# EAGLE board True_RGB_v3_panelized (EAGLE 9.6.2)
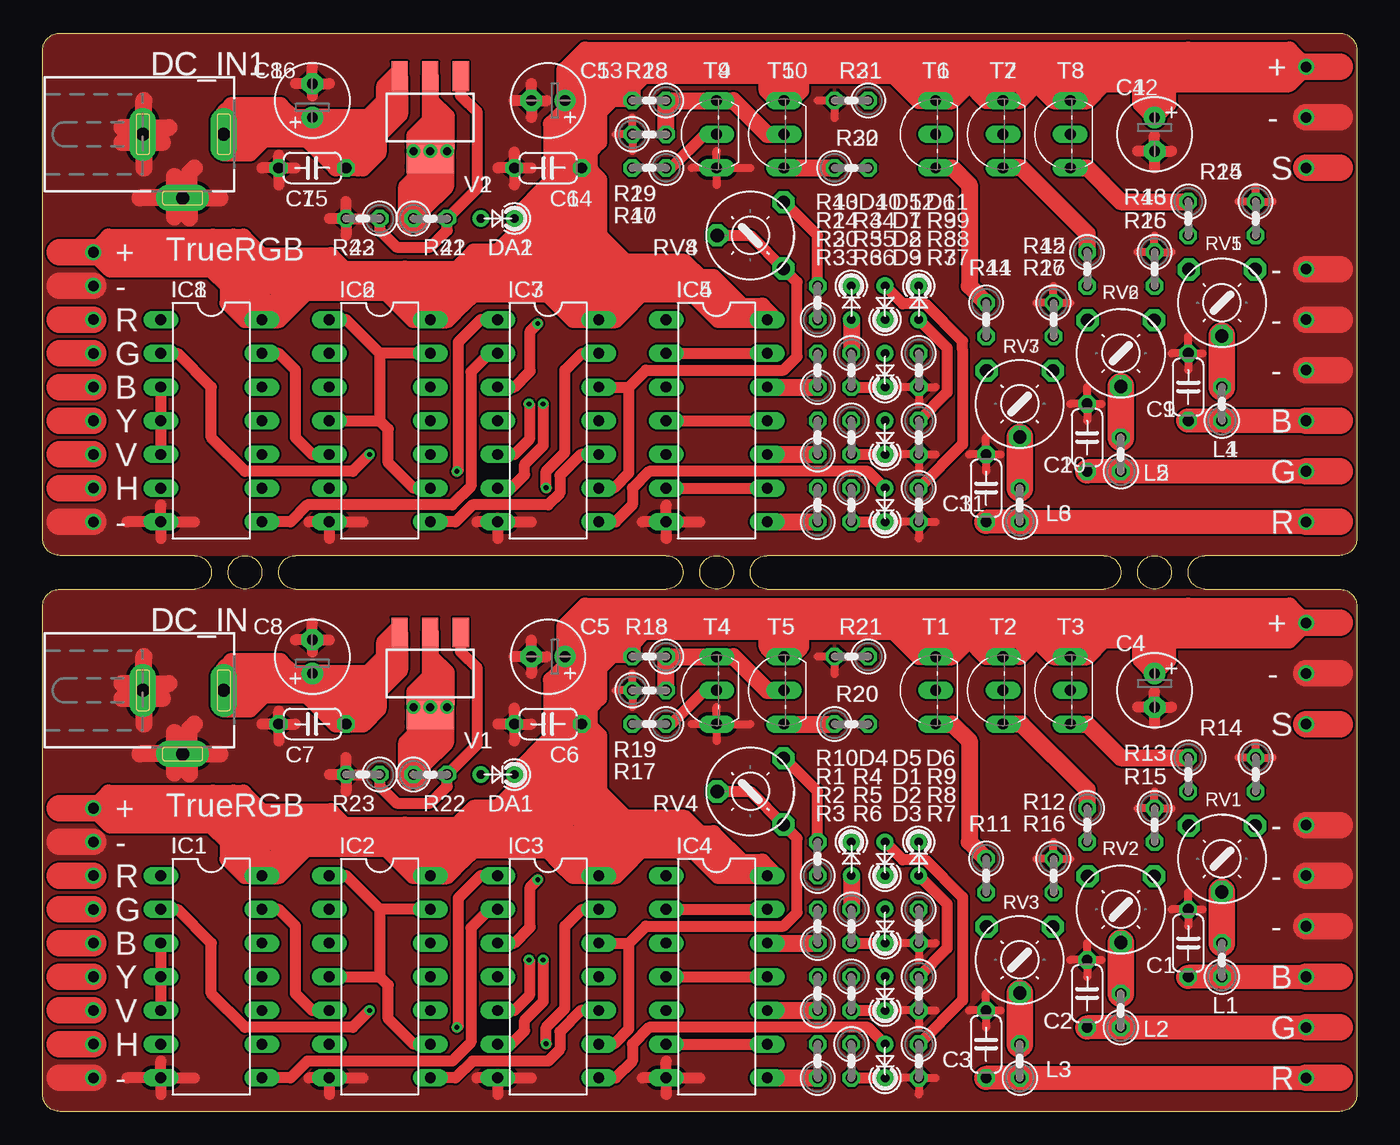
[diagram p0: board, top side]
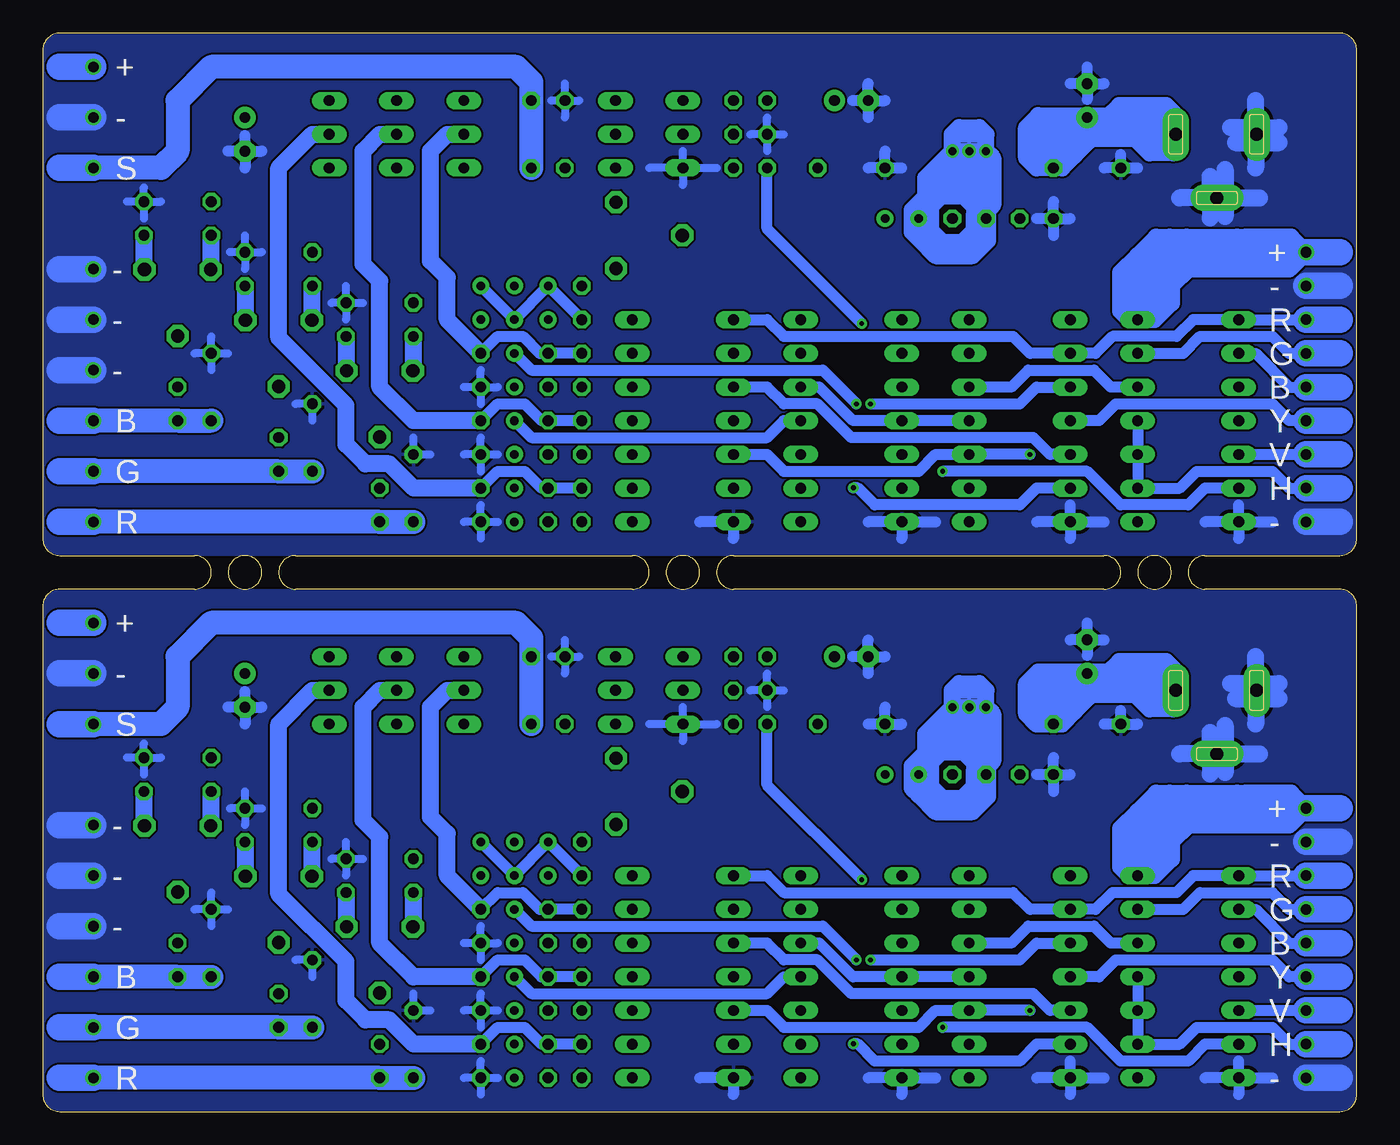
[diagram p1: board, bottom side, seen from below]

Size 99.06 x 81.28 mm. Coordinates in mm from the lower left corner, seen from the top.
Outline: 97.79,0 1.27,0 arc-90 0,1.27 0,38.1 arc-90 1.27,39.37 11.43,39.37 arc180 11.43,41.91 1.27,41.91 arc-90 0,43.18 0,80.01 arc-90 1.27,81.28 97.79,81.28 arc-90 99.06,80.01 99.06,43.18 arc-90 97.79,41.91 87.63,41.91 arc180 87.63,39.37 97.79,39.37 arc-90 99.06,38.1 99.06,1.27 arc-90 97.79,0
Outline: 19.05,39.37 46.99,39.37 arc180 46.99,41.91 19.05,41.91 arc180 19.05,39.37
Outline: 54.61,39.37 80.01,39.37 arc180 80.01,41.91 54.61,41.91 arc180 54.61,39.37
Outline: 15.24,39.37 arc-180 15.24,41.91 arc-180 15.24,39.37
Outline: 83.82,41.91 arc-180 83.82,39.37 arc-180 83.82,41.91
Outline: 50.8,41.91 arc-180 50.8,39.37 arc-180 50.8,41.91
Copper layers (1*16): Top 0.035mm / dielectric 1.5mm / Bottom 0.035mm
Design rules "default *": minimum track width 6mil, minimum drill 0.35mm, track to track 6mil, track to pad 6mil, pad to pad 6mil, via to via 6mil, smd to smd 6mil, copper to edge 2mil, drill to drill 6mil, minimum pad ring 10mil, minimum via ring 8mil, stop-mask expansion 4mil, vias tented up to drill 20mil, thermal gap 10mil
Net classes: 1 power: width 0.66 mm, clearance 0.254 mm

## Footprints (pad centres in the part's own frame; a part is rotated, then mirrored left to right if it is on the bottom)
C050-024X044 = drill 0.813 octagon: 1 -2.54,0; 2 2.54,0
E2,5-6 = drill 0.813 pad 1.6: + -1.27,0 | drill 0.813 pad 1.6 octagon: - 1.27,0
D4148-2 = drill 0.65 pad 1.27: A 1.27,0; C -1.27,0
DCJ0202 = drill 1 pad 2 long: 1 0,3.1; 2 4.8,0; 3 0,-3
DIL14 = drill 0.813 long: 1 -7.62,-3.81; 2 -5.08,-3.81; 3 -2.54,-3.81; 4 0,-3.81; 5 2.54,-3.81; 6 5.08,-3.81; 7 7.62,-3.81; 8 7.62,3.81; 9 5.08,3.81; 10 2.54,3.81; 11 0,3.81; 12 -2.54,3.81; 13 -5.08,3.81; 14 -7.62,3.81
0207/2V = drill 0.813 octagon: 1 -1.27,0; 2 1.27,0
6MM = drill 1 pad 1.676 octagon: A -2.5,-2.5; E 2.5,-2.5; S 0,2.5
TO92-EBC = drill 0.813 long: B 0,-1.27; C 2.54,-1.27; E -2.54,-1.27
SOT223 = smd 1.219 x 2.235: 1 -2.311,-3.099; 2 0,-3.099; 3 2.311,-3.099 | smd 3.6 x 2.2: TAB 0,3.099

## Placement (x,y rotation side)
C1  47  [C050-024X044]  86.36,12.7 90 top
C2  47  [C050-024X044]  78.74,8.89 90 top
C3  47  [C050-024X044]  71.12,5.08 90 top
C4  10uF  [E2,5-6]  83.82,31.75 270 top
C5  100uF  [E2,5-6]  38.1,34.29 180 top
C6  0.1uF  [C050-024X044]  38.1,29.21 180 top
C7  0.1uF  [C050-024X044]  20.32,29.21 180 top
C8  100uF  [E2,5-6]  20.32,34.29 90 top
C9  47  [C050-024X044]  86.36,54.61 90 top
C10  47  [C050-024X044]  78.74,50.8 90 top
C11  47  [C050-024X044]  71.12,46.99 90 top
C12  10uF  [E2,5-6]  83.82,73.66 270 top
C13  100uF  [E2,5-6]  38.1,76.2 180 top
C14  0.1uF  [C050-024X044]  38.1,71.12 180 top
C15  0.1uF  [C050-024X044]  20.32,71.12 180 top
C16  100uF  [E2,5-6]  20.32,76.2 90 top
D1  1N4148AS  [D4148-2]  63.5,13.97 90 top
D2  1N4148AS  [D4148-2]  63.5,8.89 90 top
D3  1N4148AS  [D4148-2]  63.5,3.81 90 top
D4  1N4148AS  [D4148-2]  60.96,19.05 270 top
D5  1N4148AS  [D4148-2]  63.5,19.05 90 top
D6  1N4148AS  [D4148-2]  66.04,19.05 270 top
D7  1N4148AS  [D4148-2]  63.5,55.88 90 top
D8  1N4148AS  [D4148-2]  63.5,50.8 90 top
D9  1N4148AS  [D4148-2]  63.5,45.72 90 top
D10  1N4148AS  [D4148-2]  60.96,60.96 270 top
D11  1N4148AS  [D4148-2]  66.04,60.96 270 top
D12  1N4148AS  [D4148-2]  63.5,60.96 90 top
DA1  BAT42  [D4148-2]  34.29,25.4 180 top
DA2  BAT42  [D4148-2]  34.29,67.31 180 top
DC_IN  DCJ0202  [DCJ0202]  10.54,31.75 270 top
DC_IN1  DCJ0202  [DCJ0202]  10.54,73.66 270 top
IC1  7427 ЛЕ4  [DIL14]  12.7,10.16 270 top
IC2  7400 ЛА3  [DIL14]  25.4,10.16 270 top
IC3  7400 ЛА3  [DIL14]  38.1,10.16 270 top
IC4  7404 ЛН1  [DIL14]  50.8,10.16 270 top
IC5  7404 ЛН1  [DIL14]  50.8,52.07 270 top
IC6  7400 ЛА3  [DIL14]  25.4,52.07 270 top
IC7  7400 ЛА3  [DIL14]  38.1,52.07 270 top
IC8  7427 ЛЕ4  [DIL14]  12.7,52.07 270 top
L1  0.56uH  [0207/2V]  88.9,11.43 90 top
L2  0.56uH  [0207/2V]  81.28,7.62 90 top
L3  0.56uH  [0207/2V]  73.66,3.81 90 top
L4  0.56uH  [0207/2V]  88.9,53.34 90 top
L5  0.56uH  [0207/2V]  81.28,49.53 90 top
L6  0.56uH  [0207/2V]  73.66,45.72 90 top
R1  2.1k  [0207/2V]  58.42,13.97 90 top
R2  2.1k  [0207/2V]  58.42,8.89 90 top
R3  2.1k  [0207/2V]  58.42,3.81 90 top
R4  330  [0207/2V]  60.96,13.97 270 top
R5  330  [0207/2V]  60.96,8.89 270 top
R6  330  [0207/2V]  60.96,3.81 270 top
R7  5.1K  [0207/2V]  66.04,3.81 270 top
R8  5.1K  [0207/2V]  66.04,8.89 270 top
R9  5.1K  [0207/2V]  66.04,13.97 270 top
R10  130  [0207/2V]  58.42,19.05 90 top
R11  100  [0207/2V]  71.12,17.78 270 top
R12  100  [0207/2V]  78.74,21.59 270 top
R13  100  [0207/2V]  86.36,25.4 270 top
R14  75  [0207/2V]  91.44,25.4 270 top
R15  75  [0207/2V]  83.82,21.59 270 top
R16  75  [0207/2V]  76.2,17.78 270 top
R17  1K  [0207/2V]  45.72,29.21 180 top
R18  1K  [0207/2V]  45.72,34.29 180 top
R19  1K  [0207/2V]  45.72,31.75 0 top
R20  47  [0207/2V]  60.96,29.21 0 top
R21  560  [0207/2V]  60.96,34.29 180 top
R22  220  [0207/2V]  29.21,25.4 0 top
R23  680  [0207/2V]  24.13,25.4 180 top
R24  2.1k  [0207/2V]  58.42,55.88 90 top
R25  75  [0207/2V]  91.44,67.31 270 top
R26  75  [0207/2V]  83.82,63.5 270 top
R27  75  [0207/2V]  76.2,59.69 270 top
R28  1K  [0207/2V]  45.72,76.2 180 top
R29  1K  [0207/2V]  45.72,73.66 0 top
R30  2.1k  [0207/2V]  58.42,50.8 90 top
R31  560  [0207/2V]  60.96,76.2 180 top
R32  47  [0207/2V]  60.96,71.12 0 top
R33  2.1k  [0207/2V]  58.42,45.72 90 top
R34  330  [0207/2V]  60.96,55.88 270 top
R35  330  [0207/2V]  60.96,50.8 270 top
R36  330  [0207/2V]  60.96,45.72 270 top
R37  5.1K  [0207/2V]  66.04,45.72 270 top
R38  5.1K  [0207/2V]  66.04,50.8 270 top
R39  5.1K  [0207/2V]  66.04,55.88 270 top
R40  1K  [0207/2V]  45.72,71.12 180 top
R41  220  [0207/2V]  29.21,67.31 0 top
R42  680  [0207/2V]  24.13,67.31 180 top
R43  130  [0207/2V]  58.42,60.96 90 top
R44  100  [0207/2V]  71.12,59.69 270 top
R45  100  [0207/2V]  78.74,63.5 270 top
R46  100  [0207/2V]  86.36,67.31 270 top
RV1  200  [6MM]  88.9,19.05 180 top
RV2  200  [6MM]  81.28,15.24 180 top
RV3  200  [6MM]  73.66,11.43 180 top
RV4  200  [6MM]  53.34,24.13 90 top
RV5  200  [6MM]  88.9,60.96 180 top
RV6  200  [6MM]  81.28,57.15 180 top
RV7  200  [6MM]  73.66,53.34 180 top
RV8  200  [6MM]  53.34,66.04 90 top
T1  4401  [TO92-EBC]  66.04,31.75 90 top
T2  4401  [TO92-EBC]  71.12,31.75 90 top
T3  4401  [TO92-EBC]  76.2,31.75 90 top
T4  4401  [TO92-EBC]  49.53,31.75 90 top
T5  4401  [TO92-EBC]  54.61,31.75 90 top
T6  4401  [TO92-EBC]  66.04,73.66 90 top
T7  4401  [TO92-EBC]  71.12,73.66 90 top
T8  4401  [TO92-EBC]  76.2,73.66 90 top
T9  4401  [TO92-EBC]  49.53,73.66 90 top
T10  4401  [TO92-EBC]  54.61,73.66 90 top
V1  LM1117IMPX-ADJ  [SOT223]  29.21,33.02 180 top
V2  LM1117IMPX-ADJ  [SOT223]  29.21,74.93 180 top

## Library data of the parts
C1-C16 = rcl; SPICEPREFIX: C
D1-D12 DA1 DA2 RV1-RV8 = 27C322
DC_IN DC_IN1 = power_jack; OC_FARNELL: unknown; OC_NEWARK: unknown
IC1-IC8 = 74xx-eu
L1-L6 = rcl; SPICEPREFIX: L
R1-R46 = rcl; SPICEPREFIX: R
T1-T10 = transistor-neu-to92
V1 V2 = lm1117

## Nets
B: IC1.2 IC2.10 IC4.5
B1: IC5.5 IC6.10 IC8.2
BLUE: C1.1 L1.1
BLUE1: C9.1 L4.1
G: IC1.13 IC2.5 IC4.3
G1: IC5.3 IC6.5 IC8.13
GND: C1.2 C2.2 C3.2 C4.- C5.- C6.2 C7.2 C8.- DC_IN.2 DC_IN.3 IC1.7 IC2.7 IC3.7 IC4.7 R7.2 R8.2 R9.2 R14.1 R15.1 R16.1 R19.1 R21.2 R23.2 T4.E
GND1: C9.2 C10.2 C11.2 C12.- C13.- C14.2 C15.2 C16.- DC_IN1.2 DC_IN1.3 IC5.7 IC6.7 IC7.7 IC8.7 R25.1 R26.1 R27.1 R29.1 R31.2 R37.2 R38.2 R39.2 R42.2 T9.E
GREEN: C2.1 L2.1
GREEN1: C10.1 L5.1
H: IC1.9 IC1.10 IC1.11
H1: IC8.9 IC8.10 IC8.11
N$1: D3.C R6.2
N$2: D2.C R5.2
N$3: D1.C R4.2
N$4: L1.2 RV1.S
N$5: IC1.12 IC2.12
N$6: IC1.8 IC3.2
N$7: L2.2 RV2.S
N$8: D5.A R3.2 R6.1 R7.1 T3.B
N$9: D6.A R2.2 R5.1 R8.1 T2.B
N$10: D4.A R1.2 R4.1 R9.1 T1.B
N$11: L3.2 RV3.S
N$12: R14.2 RV1.A
N$13: R15.2 RV2.A
N$14: R16.2 RV3.A
N$15: R11.1 T1.E
N$16: R12.2 RV2.E
N$17: R11.2 RV3.E
N$18: R12.1 T2.E
N$19: IC2.3 IC3.5
N$20: IC2.6 IC3.13
N$21: IC2.8 IC3.10
N$22: D1.A IC3.6
N$23: D2.A IC3.11
N$24: D3.A IC3.8
N$25: IC4.2 IC4.13
N$26: IC4.4 IC4.11
N$27: IC4.6 IC4.9
N$28: IC4.12 R1.1
N$29: IC4.10 R2.1
N$30: IC4.8 R3.1
N$31: IC3.3 R17.2
N$32: R22.2 R23.1 V1.1
N$33: IC1.6 IC3.1
N$34: R17.1 T4.B
N$35: DA1.A R22.1 V1.2 V1.TAB
N$36: D4.C D5.C D6.C R10.1
N$37: R10.2 RV4.E
N$38: IC2.11 IC3.4 IC3.9 IC3.12 RV4.A RV4.S
N$39: R13.1 T3.E
N$40: R13.2 RV1.E
N$41: D12.A R33.2 R36.1 R37.1 T8.B
N$42: D11.A R30.2 R35.1 R38.1 T7.B
N$43: D10.A R24.2 R34.1 R39.1 T6.B
N$44: R28.1 R29.2 T9.C T10.B
N$45: R32.1 T10.E
N$46: L4.2 RV5.S
N$47: L5.2 RV6.S
N$48: L6.2 RV7.S
N$49: R25.2 RV5.A
N$50: R26.2 RV6.A
N$51: R27.2 RV7.A
N$52: R45.2 RV6.E
N$53: R44.2 RV7.E
N$54: IC6.3 IC7.5
N$55: IC6.6 IC7.13
N$56: IC6.8 IC7.10
N$57: D7.A IC7.6
N$58: D8.A IC7.11
N$59: D9.A IC7.8
N$60: IC5.2 IC5.13
N$61: IC5.4 IC5.11
N$62: IC5.6 IC5.9
N$63: IC5.12 R24.1
N$64: IC5.10 R30.1
N$65: IC5.8 R33.1
N$66: D9.C R36.2
N$67: D8.C R35.2
N$68: D7.C R34.2
N$69: IC6.12 IC8.12
N$70: IC7.3 R40.2
N$71: R40.1 T9.B
N$72: DA2.A R41.1 V2.2 V2.TAB
N$73: R41.2 R42.1 V2.1
N$74: IC7.2 IC8.8
N$75: IC7.1 IC8.6
N$76: D10.C D11.C D12.C R43.1
N$77: IC6.11 IC7.4 IC7.9 IC7.12 RV8.A RV8.S
N$78: R44.1 T6.E
N$79: R45.1 T7.E
N$80: R46.1 T8.E
N$81: R46.2 RV5.E
N$82: R43.2 RV8.E
N$176: R20.1 T5.E
N$177: R18.1 R19.2 T4.C T5.B
R: IC1.1 IC2.2 IC4.1
R1: IC5.1 IC6.2 IC8.1
RED: C3.1 L3.1
RED1: C11.1 L6.1
S: R20.2 R21.1
S1: R31.1 R32.2
V: IC1.3 IC1.4 IC1.5
V1: IC8.3 IC8.4 IC8.5
VCC: C4.+ C5.+ C6.1 DA1.C IC1.14 IC2.14 IC3.14 IC4.14 R18.2 T1.C T2.C T3.C T5.C
VCC1: C12.+ C13.+ C14.1 DA2.C IC5.14 IC6.14 IC7.14 IC8.14 R28.2 T6.C T7.C T8.C T10.C
VIN: C7.1 C8.+ DC_IN.1 V1.3
VIN1: C15.1 C16.+ DC_IN1.1 V2.3
Y: IC2.1 IC2.4 IC2.9 IC2.13
Y1: IC6.1 IC6.4 IC6.9 IC6.13

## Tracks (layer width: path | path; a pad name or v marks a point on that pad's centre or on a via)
B  (via drill 0.35, 0.8)
  Top 0.813: IC1.2 10.16,15.24 12.7,12.7 12.7,8.89 15.24,6.35 23.37,6.35 v24.64,7.62
  Top 2: v3.81,12.7 1.27,12.7
  Bottom 0.813: v24.64,7.62 IC2.10 31.75,7.62 33.02,6.35 43.18,6.35 44.45,7.62 IC4.5 | IC1.2 7.62,15.24 5.08,12.7 v3.81,12.7
  Bottom 2: 1.27,12.7 v3.81,12.7
B1  (via drill 0.35, 0.8)
  Top 0.813: IC8.2 10.16,57.15 12.7,54.61 12.7,50.8 15.24,48.26 23.37,48.26 v24.64,49.53
  Top 2: v3.81,54.61 1.27,54.61
  Bottom 0.813: v24.64,49.53 IC6.10 31.75,49.53 33.02,48.26 43.18,48.26 44.45,49.53 IC5.5 | IC8.2 7.62,57.15 5.08,54.61 v3.81,54.61
  Bottom 2: 1.27,54.61 v3.81,54.61
BLUE  (via drill 0.8)
  Top 1.8: v95.25,10.16 L1.1 C1.1
  Top 2: v95.25,10.16 97.79,10.16
  Bottom 1.8: v95.25,10.16 L1.1 C1.1
  Bottom 2: v95.25,10.16 97.79,10.16
BLUE1  (via drill 0.8)
  Top 1.8: v95.25,52.07 L4.1 C9.1
  Top 2: v95.25,52.07 97.79,52.07
  Bottom 1.8: v95.25,52.07 L4.1 C9.1
  Bottom 2: v95.25,52.07 97.79,52.07
G  (via drill 0.8)
  Top 0.813: IC2.5 20.32,7.62 19.05,8.89 19.05,13.97 17.78,15.24 IC1.13
  Top 2: v3.81,15.24 1.27,15.24
  Bottom 0.813: IC2.5 23.11,7.62 24.38,8.89 38.1,8.89 40.64,11.43 43.18,11.43 44.45,12.7 IC4.3 | IC1.13 13.08,15.24 11.81,16.51 6.35,16.51 5.08,15.24 v3.81,15.24
  Bottom 2: 1.27,15.24 v3.81,15.24
G1  (via drill 0.8)
  Top 0.813: IC6.5 20.32,49.53 19.05,50.8 19.05,55.88 17.78,57.15 IC8.13
  Top 2: v3.81,57.15 1.27,57.15
  Bottom 0.813: IC6.5 23.11,49.53 24.38,50.8 38.1,50.8 40.64,53.34 43.18,53.34 44.45,54.61 IC5.3 | IC8.13 13.08,57.15 11.81,58.42 6.35,58.42 5.08,57.15 v3.81,57.15
  Bottom 2: 1.27,57.15 v3.81,57.15
GND  (via drill 0.8)
  Top 0.61: R14.1 92.71,26.67 | R14.1 91.44,27.81 | R14.1 90.17,26.67 | R14.1 91.44,25.4 | R15.1 83.82,24.13 | R15.1 85.09,22.86 | R15.1 82.55,22.86 | R15.1 83.82,21.59 | C1.2 86.36,16.51 | C1.2 85.09,15.24 | C1.2 86.36,13.97 | C1.2 87.44,15.24 | R16.1 76.2,20.32 | R16.1 76.2,17.78 | R16.1 74.93,19.05 | R16.1 77.47,19.05 | R9.2 67.31,12.7 | R9.2 66.04,13.97 | R9.2 64.77,12.7 | R9.2 66.04,11.43 | R8.2 67.31,7.62 | R8.2 66.04,8.89 | R8.2 64.77,7.62 | R8.2 66.04,6.35 | R7.2 67.31,2.54 | R7.2 66.04,3.81 | R7.2 64.77,2.54 | R7.2 66.04,1.27 | C3.2 71.12,8.89 | C3.2 71.12,6.35 | C3.2 69.85,7.62 | C3.2 72.2,7.62 | C2.2 78.74,10.16 | C2.2 78.74,12.7 | C2.2 79.82,11.43 | C2.2 77.47,11.43 | T4.E 50.8,27.94 | T4.E 48.92,29.21 | T4.E 53.34,29.21 | T4.E 50.8,30.48 | R21.2 59.69,32.97 | R21.2 58.42,34.29 | R21.2 60.96,34.29 | R19.1 43.18,31.75 | R19.1 44.45,33.02 | R19.1 44.45,30.48 | R19.1 45.72,31.75
  Top 0.813: C5.- 36.83,35.56 | C5.- 35.56,34.29 | C5.- 38.01,34.29 | C5.- 36.83,33.02 | C6.2 35.56,30.43 | C6.2 34.29,29.21 | C6.2 36.83,29.21 | C6.2 35.56,27.94 | C8.- 20.32,36.83 | C8.- 21.59,35.56 | C8.- 19.05,35.56 | C8.- 20.32,34.63 | C7.2 19.05,29.21 | C7.2 16.51,29.21 | C7.2 17.78,30.18 | C7.2 17.78,27.94 | IC1.7 11.43,2.54 | IC1.7 6.35,2.54 | IC1.7 8.89,3.81 | IC1.7 8.89,1.27 | IC2.7 20.07,2.54 | IC2.7 24.13,2.54 | IC2.7 21.59,1.27 | IC3.7 32.73,2.54 | IC3.7 36.83,2.54 | IC3.7 34.29,1.27 | IC4.7 45.21,2.54 | IC4.7 46.99,3.81 | IC4.7 46.99,1.27 | IC4.7 49.53,2.54 | C4.- 83.82,31.66 | C4.- 83.82,29.21 | C4.- 85.09,30.48 | C4.- 82.55,30.48 | R23.2 22.86,26.67 | R23.2 21.59,25.4 | R23.2 24.13,25.4 | R23.2 22.86,24.13
  Top 1.27: DC_IN.3 8.18,31.11 9.02,31.11 | DC_IN.3 6.91,31.11 5.97,31.11 | DC_IN.3 7.62,31.83 7.62,34.29 | DC_IN.3 7.62,31.67 7.62,29.21 | 9.91,28.57 9.91,27.59 DC_IN.2 | DC_IN.2 9.91,26.32 9.91,25.53 | DC_IN.2 7.34,26.95 | DC_IN.2 13.36,26.95 | DC_IN.2 11.05,27.46 11.05,28.83 11.43,29.21 | DC_IN.2 11.05,26.44 11.05,25.43 | DC_IN.3 7.03,32.26 5.97,32.26 | DC_IN.3 8.05,32.26 9.53,32.26
  Top 2: v3.81,2.54 1.27,2.54 | v95.25,21.59 97.79,21.59 | v95.25,17.78 97.79,17.78 | v95.25,13.97 97.79,13.97 | v95.25,33.02 97.79,33.02 | v3.81,20.32 1.27,20.32
  Bottom 0.61: R19.1 44.45,33.02 | R19.1 43.18,31.75 | R19.1 45.72,31.75 | R19.1 44.45,30.48 | T4.E 48.26,29.21 | T4.E 50.8,30.48 | T4.E 50.8,27.94 | T4.E 53.34,29.21 | R21.2 60.71,34.29 | R21.2 59.69,33.02 | R21.2 58.61,34.29 | R21.2 59.69,35.56 | 78.74,10.16 C2.2 80.01,11.43 | C1.2 86.36,16.51 | C1.2 85.09,15.24 | C1.2 87.63,15.24 | C1.2 86.36,13.97 | 71.12,8.89 C3.2 69.85,7.62 | R8.2 66.04,8.89 | R8.2 64.77,7.62 | R8.2 67.31,7.62 | R8.2 66.04,6.35 | R7.2 66.04,1.27 | R7.2 67.31,2.54 | R7.2 64.77,2.54 | R7.2 66.04,3.81 | R9.2 66.04,13.97 | R9.2 67.31,12.7 | R9.2 64.77,12.7 | R9.2 66.04,11.43 | R16.1 76.2,20.32 | R16.1 74.93,19.05 | R16.1 76.2,17.78 | R16.1 77.32,19.05 | R15.1 83.82,24.13 | R15.1 83.82,21.59 | R15.1 84.94,22.86 | R15.1 82.55,22.86 | R14.1 91.44,27.75 | R14.1 92.71,26.67 | R14.1 90.17,26.67 | R14.1 91.44,25.4
  Bottom 0.813: C7.2 17.78,30.23 | C7.2 19.05,29.21 | C7.2 16.51,29.21 | C8.- 20.32,36.83 | C8.- 20.32,34.38 | C8.- 21.59,35.56 | C8.- 19.05,35.56 | C6.2 34.29,29.21 | C6.2 36.83,29.21 | C6.2 35.56,30.48 | C5.- 36.83,35.56 | C5.- 38.01,34.29 | C5.- 35.56,34.29 | C5.- 36.83,33.02 | C4.- 82.55,30.48 | C4.- 83.82,29.21 | C4.- 85.09,30.48 | C4.- 83.82,31.66 | IC1.7 11.43,2.54 | IC1.7 8.89,3.81 | IC1.7 8.89,1.27 | IC2.7 19.05,2.54 | IC2.7 21.59,3.81 | IC2.7 21.59,1.27 | IC2.7 24.13,2.54 | IC3.7 31.75,2.54 | IC3.7 36.83,2.54 | IC3.7 34.29,1.27 | 49.53,2.54 IC4.7 46.99,1.27 | IC1.7 6.35,2.54 | R23.2 21.59,25.4 | R23.2 22.86,26.67 | R23.2 22.86,24.13 | R23.2 24.13,25.4
  Bottom 1.27: DC_IN.3 7.62,31.83 7.62,34.29 | DC_IN.3 7.62,31.67 7.62,29.21 | DC_IN.3 8.18,31.11 9.14,31.11 | DC_IN.3 6.91,31.11 5.84,31.11 | DC_IN.2 7.34,26.95 | DC_IN.2 9.91,27.59 9.91,29.08 | DC_IN.2 9.91,26.32 9.91,25.55 | DC_IN.2 13.36,26.95 | DC_IN.2 11.05,27.46 11.05,28.57 | DC_IN.2 11.05,26.44 11.05,25.43 | DC_IN.3 7.03,32.26 5.84,32.26 | DC_IN.3 8.05,32.26 9.53,32.26
  Bottom 2: v3.81,2.54 1.27,2.54 | v95.25,33.02 97.79,33.02 | v95.25,21.59 97.79,21.59 | v95.25,17.78 97.79,17.78 | v95.25,13.97 97.79,13.97 | v3.81,20.32 1.27,20.32
  pour Bottom: 0,39.37 99.06,39.37 99.06,0 0,0
  pour Top: 0,39.37 99.06,39.37 99.06,0 0,0
GND1  (via drill 0.8)
  Top 0.61: R25.1 92.71,68.58 | R25.1 91.44,69.72 | R25.1 90.17,68.58 | R25.1 91.44,67.31 | R26.1 83.82,66.04 | R26.1 85.09,64.77 | R26.1 82.55,64.77 | R26.1 83.82,63.5 | C9.2 86.36,58.42 | C9.2 85.09,57.15 | C9.2 86.36,55.88 | C9.2 87.44,57.15 | R27.1 76.2,62.23 | R27.1 76.2,59.69 | R27.1 74.93,60.96 | R27.1 77.47,60.96 | R39.2 67.31,54.61 | R39.2 66.04,55.88 | R39.2 64.77,54.61 | R39.2 66.04,53.34 | R38.2 67.31,49.53 | R38.2 66.04,50.8 | R38.2 64.77,49.53 | R38.2 66.04,48.26 | R37.2 67.31,44.45 | R37.2 66.04,45.72 | R37.2 64.77,44.45 | R37.2 66.04,43.18 | C11.2 71.12,50.8 | C11.2 71.12,48.26 | C11.2 69.85,49.53 | C11.2 72.2,49.53 | C10.2 78.74,52.07 | C10.2 78.74,54.61 | C10.2 79.82,53.34 | C10.2 77.47,53.34 | T9.E 50.8,69.85 | T9.E 48.92,71.12 | T9.E 53.34,71.12 | T9.E 50.8,72.39 | R31.2 59.69,74.88 | R31.2 58.42,76.2 | R31.2 60.96,76.2 | R29.1 43.18,73.66 | R29.1 44.45,74.93 | R29.1 44.45,72.39 | R29.1 45.72,73.66
  Top 0.813: C13.- 36.83,77.47 | C13.- 35.56,76.2 | C13.- 38.01,76.2 | C13.- 36.83,74.93 | C14.2 35.56,72.34 | C14.2 34.29,71.12 | C14.2 36.83,71.12 | C14.2 35.56,69.85 | C16.- 20.32,78.74 | C16.- 21.59,77.47 | C16.- 19.05,77.47 | C16.- 20.32,76.54 | C15.2 19.05,71.12 | C15.2 16.51,71.12 | C15.2 17.78,72.08 | C15.2 17.78,69.85 | IC8.7 11.43,44.45 | IC8.7 6.35,44.45 | IC8.7 8.89,45.72 | IC8.7 8.89,43.18 | IC6.7 20.07,44.45 | IC6.7 24.13,44.45 | IC6.7 21.59,43.18 | IC7.7 32.73,44.45 | IC7.7 36.83,44.45 | IC7.7 34.29,43.18 | IC5.7 45.21,44.45 | IC5.7 46.99,45.72 | IC5.7 46.99,43.18 | IC5.7 49.53,44.45 | C12.- 83.82,73.57 | C12.- 83.82,71.12 | C12.- 85.09,72.39 | C12.- 82.55,72.39 | R42.2 22.86,68.58 | R42.2 21.59,67.31 | R42.2 24.13,67.31 | R42.2 22.86,66.04
  Top 1.27: DC_IN1.3 8.18,73.03 9.02,73.03 | DC_IN1.3 6.91,73.03 5.97,73.03 | DC_IN1.3 7.62,73.74 7.62,76.2 | DC_IN1.3 7.62,73.58 7.62,71.12 | 9.91,70.48 9.91,69.5 DC_IN1.2 | DC_IN1.2 9.91,68.22 9.91,67.44 | DC_IN1.2 7.34,68.86 | DC_IN1.2 13.36,68.86 | DC_IN1.2 11.05,69.37 11.05,70.74 11.43,71.12 | DC_IN1.2 11.05,68.35 11.05,67.33 | DC_IN1.3 7.03,74.17 5.97,74.17 | DC_IN1.3 8.05,74.17 9.53,74.17
  Top 2: v3.81,44.45 1.27,44.45 | v95.25,63.5 97.79,63.5 | v95.25,59.69 97.79,59.69 | v95.25,55.88 97.79,55.88 | v95.25,74.93 97.79,74.93 | v3.81,62.23 1.27,62.23
  Bottom 0.61: R29.1 44.45,74.93 | R29.1 43.18,73.66 | R29.1 45.72,73.66 | R29.1 44.45,72.39 | T9.E 48.26,71.12 | T9.E 50.8,72.39 | T9.E 50.8,69.85 | T9.E 53.34,71.12 | R31.2 60.71,76.2 | R31.2 59.69,74.93 | R31.2 58.61,76.2 | R31.2 59.69,77.47 | 78.74,52.07 C10.2 80.01,53.34 | C9.2 86.36,58.42 | C9.2 85.09,57.15 | C9.2 87.63,57.15 | C9.2 86.36,55.88 | 71.12,50.8 C11.2 69.85,49.53 | R38.2 66.04,50.8 | R38.2 64.77,49.53 | R38.2 67.31,49.53 | R38.2 66.04,48.26 | R37.2 66.04,43.18 | R37.2 67.31,44.45 | R37.2 64.77,44.45 | R37.2 66.04,45.72 | R39.2 66.04,55.88 | R39.2 67.31,54.61 | R39.2 64.77,54.61 | R39.2 66.04,53.34 | R27.1 76.2,62.23 | R27.1 74.93,60.96 | R27.1 76.2,59.69 | R27.1 77.32,60.96 | R26.1 83.82,66.04 | R26.1 83.82,63.5 | R26.1 84.94,64.77 | R26.1 82.55,64.77 | R25.1 91.44,69.66 | R25.1 92.71,68.58 | R25.1 90.17,68.58 | R25.1 91.44,67.31
  Bottom 0.813: C15.2 17.78,72.14 | C15.2 19.05,71.12 | C15.2 16.51,71.12 | C16.- 20.32,78.74 | C16.- 20.32,76.29 | C16.- 21.59,77.47 | C16.- 19.05,77.47 | C14.2 34.29,71.12 | C14.2 36.83,71.12 | C14.2 35.56,72.39 | C13.- 36.83,77.47 | C13.- 38.01,76.2 | C13.- 35.56,76.2 | C13.- 36.83,74.93 | C12.- 82.55,72.39 | C12.- 83.82,71.12 | C12.- 85.09,72.39 | C12.- 83.82,73.57 | IC8.7 11.43,44.45 | IC8.7 8.89,45.72 | IC8.7 8.89,43.18 | IC6.7 19.05,44.45 | IC6.7 21.59,45.72 | IC6.7 21.59,43.18 | IC6.7 24.13,44.45 | IC7.7 31.75,44.45 | IC7.7 36.83,44.45 | IC7.7 34.29,43.18 | 49.53,44.45 IC5.7 46.99,43.18 | IC8.7 6.35,44.45 | R42.2 21.59,67.31 | R42.2 22.86,68.58 | R42.2 22.86,66.04 | R42.2 24.13,67.31
  Bottom 1.27: DC_IN1.3 7.62,73.74 7.62,76.2 | DC_IN1.3 7.62,73.58 7.62,71.12 | DC_IN1.3 8.18,73.03 9.14,73.03 | DC_IN1.3 6.91,73.03 5.84,73.03 | DC_IN1.2 7.34,68.86 | DC_IN1.2 9.91,69.5 9.91,70.99 | DC_IN1.2 9.91,68.22 9.91,67.46 | DC_IN1.2 13.36,68.86 | DC_IN1.2 11.05,69.37 11.05,70.48 | DC_IN1.2 11.05,68.35 11.05,67.33 | DC_IN1.3 7.03,74.17 5.84,74.17 | DC_IN1.3 8.05,74.17 9.53,74.17
  Bottom 2: v3.81,44.45 1.27,44.45 | v95.25,74.93 97.79,74.93 | v95.25,63.5 97.79,63.5 | v95.25,59.69 97.79,59.69 | v95.25,55.88 97.79,55.88 | v3.81,62.23 1.27,62.23
  pour Bottom: 0,81.28 99.06,81.28 99.06,41.91 0,41.91
  pour Top: 0,81.28 99.06,81.28 99.06,41.91 0,41.91
GREEN  (via drill 0.8)
  Top 1.8: v95.25,6.35 L2.1 C2.1
  Top 2: 97.79,6.35 v95.25,6.35
  Bottom 1.8: v95.25,6.35 L2.1 C2.1
  Bottom 2: v95.25,6.35 97.79,6.35
GREEN1  (via drill 0.8)
  Top 1.8: v95.25,48.26 L5.1 C10.1
  Top 2: 97.79,48.26 v95.25,48.26
  Bottom 1.8: v95.25,48.26 L5.1 C10.1
  Bottom 2: v95.25,48.26 97.79,48.26
H  (via drill 0.8)
  Top 2: v3.81,5.08 1.27,5.08
  Bottom 0.813: v3.81,5.08 5.08,5.08 6.35,6.35 12.06,6.35 13.34,5.08 IC1.9 IC1.10 IC1.11
  Bottom 2: v3.81,5.08 1.27,5.08
H1  (via drill 0.8)
  Top 2: v3.81,46.99 1.27,46.99
  Bottom 0.813: v3.81,46.99 5.08,46.99 6.35,48.26 12.06,48.26 13.34,46.99 IC8.9 IC8.10 IC8.11
  Bottom 2: v3.81,46.99 1.27,46.99
N$1
  Top 0.813: R6.2 D3.C
N$2
  Top 0.813: R5.2 D2.C
N$3
  Top 0.813: R4.2 D1.C
N$4
  Top 2: RV1.S L1.2
N$5
  Bottom 0.813: IC1.12 18.54,12.7 19.81,13.97 24.77,13.97 26.03,12.7 IC2.12
N$6
  Top 0.813: IC3.2 33.68,15.24 32.28,13.84 32.28,5.23 30.86,3.81 19.94,3.81 18.67,2.54 IC1.8
N$7
  Top 2: RV2.S L2.2
N$8
  Top 0.813: R7.1 69.34,8.38 69.34,16.17 66.53,18.97 64.85,18.97 D5.A
  Bottom 0.813: R3.2 R6.1 61.47,5.08 62.74,6.35 64.77,6.35 R7.1
  Bottom 1.27: R7.1 71.1,5.08 72.93,6.91 74.73,6.91 76.2,8.38 76.2,11.31 81.28,16.39 81.28,29.21 78.74,31.75 T3.B
N$9
  Top 0.813: R8.1 68.17,12.29 68.17,15.65 D6.A
  Bottom 0.813: R2.2 R5.1 61.47,10.16 62.74,11.43 64.77,11.43 R8.1
  Bottom 1.27: R8.1 71.12,10.16 73.66,12.7 73.66,20.7 74.93,21.97 74.93,30.48 73.66,31.75 T2.B
N$10
  Top 1.27: D4.A R4.1
  Bottom 0.813: R1.2 R4.1 61.59,15.24 62.87,16.51 64.77,16.51 R9.1
  Bottom 1.27: R9.1 68.58,17.78 68.58,20.95 69.83,22.2 69.83,30.5 68.58,31.75 T1.B
N$11
  Top 2: RV3.S L3.2
N$12
  Bottom 1.27: R14.2 91.44,21.59 RV1.A
N$13
  Bottom 1.27: R15.2 83.82,17.78 RV2.A
N$14
  Bottom 1.27: R16.2 76.2,13.97 RV3.A
N$15
  Top 1.27: T1.E 68.58,29.21 69.85,27.94 69.85,20.32 R11.1
N$16
  Bottom 1.27: R12.2 78.78,20.28 RV2.E
N$17
  Bottom 1.27: R11.2 71.16,16.47 RV3.E
N$18
  Top 1.27: R12.1 78.74,24.26 73.79,29.21 T2.E
N$19  (via drill 0.35)
  Top 0.813: IC3.5 35.56,7.62 36.69,8.75 36.69,11.39 v36.66,11.43
  Bottom 0.813: v36.66,11.43 25.4,11.43 24.13,12.7 IC2.3
N$20  (via drill 0.35)
  Top 0.813: v37.95,5.11 37.95,6.35 39.37,7.78 39.37,13.97 40.64,15.24 IC3.13
  Bottom 0.813: IC2.6 24.13,5.08 25.4,3.81 36.32,3.81 37.62,5.11 v37.95,5.11
N$21
  Top 0.813: IC3.10 40.58,7.62 38.99,6.03 38.99,4.7 38.1,3.81 32.39,3.81 31.12,2.54 IC2.8
N$22  (via drill 0.35)
  Top 0.813: IC3.6 35.31,5.08 36.32,6.1 36.32,6.89 37.72,8.29 v37.72,11.43
  Bottom 0.813: v37.72,11.43 40.26,13.97 62.23,13.97 D1.A
N$23
  Bottom 0.813: D2.A 62.23,8.89 44.45,8.89 43.18,10.16 IC3.11
N$24
  Top 0.813: D3.A 62.23,6.35 45.72,6.35 44.45,5.08 44.45,3.81 43.18,2.54 IC3.8
N$25
  Top 0.813: IC4.2 IC4.13
N$26
  Top 0.813: IC4.4 IC4.11
N$27
  Top 0.813: IC4.6 IC4.9
N$28
  Top 1.27: IC4.12 R1.1
N$29
  Top 1.27: IC4.10 R2.1
N$30
  Top 1.27: IC4.8 R3.1
N$31  (via drill 0.35)
  Top 0.813: IC3.3 35.56,12.7 36.75,13.89 36.75,16.92 v37.31,17.48
  Bottom 0.813: v37.31,17.48 44.45,24.61 R17.2
N$32
  Top 0.813: V1.1 31.5,36.09 31.5,34.67 32.77,33.4 32.77,27.69 R22.2 30.48,24.51 29.21,23.24 26.67,23.24 25.4,24.51 R23.1
N$33  (via drill 0.35)
  Top 0.813: IC3.1 33.02,17.78 31.32,16.08 31.32,6.45 v31.22,6.35
  Bottom 0.813: IC1.6 11.43,5.08 12.7,3.81 17.78,3.81 20.32,6.35 v31.22,6.35
N$34
  Top 0.813: R17.1 47.37,29.21 49.91,31.75 T4.B
N$35  (via drill 0.6)
  Top 1.27: V1.2 29.21,34.29 | 29.21,34.29 29.21,32.77 | 29.21,32.77 v29.21,30.48 | v29.21,30.48 V1.TAB | V1.TAB 28.07,31.06 28.07,31.62 29.21,32.77 | 29.21,34.29 30.43,33.07 30.43,30.76 29.59,29.92 V1.TAB | v29.21,30.48 28.07,29.34 28.07,28.45 | 28.07,28.45 28.07,26.67 | 28.07,26.67 28.07,25.53 | 27.43,25.4 R22.1 28.07,25.53 | 28.07,28.45 27.43,27.81 27.43,25.4 | 28.07,25.53 29.21,26.67 V1.TAB | V1.TAB 30.35,29.92 30.35,27.81 28.7,26.16 | 28.7,26.16 28.45,25.91 28.45,25.15 28.19,24.89 27.69,24.89 27.43,25.15 27.43,25.4 | 28.07,26.67 28.7,26.67 28.7,26.16
  Bottom 1.27: DA1.A 33.02,26.54 | 32.51,27.05 31.62,27.94 31.62,29.34 | 31.62,29.34 v30.48,30.48 | v30.48,30.48 v29.21,30.48 | v29.21,30.48 v27.94,30.48 | v27.94,30.48 27.43,29.97 27.43,26.42 27.81,26.04 27.81,25.4 | 27.81,25.4 R22.1 | R22.1 28.43,25.4 28.82,25.79 | 30.48,27.1 31.32,27.1 DA1.A | R22.1 27.94,28.83 29.21,30.1 v29.21,30.48 | v29.21,30.48 29.08,30.34 29.08,26.67 | 29.08,26.67 29.08,26.54 29.63,27.1 | 28.82,25.79 28.82,26.42 29.08,26.67 | v30.48,30.48 30.48,27.1 | 30.48,27.1 29.63,27.1 | 29.63,27.1 29.51,27.1 29.72,27.31 29.72,29.97 v29.21,30.48 | v30.48,30.48 30.48,31.75 | 30.48,31.75 29.97,32.26 28.45,32.26 27.94,31.75 | v27.94,30.48 27.94,31.75 | 27.94,31.75 30.48,31.75 | 31.62,29.34 32.51,28.45 32.51,27.05 | 32.51,27.05 33.02,26.54 | DA1.A 32.13,26.29 32.13,24.51 31.24,23.62 29.72,23.62 28.82,24.52 28.82,25.79 | 27.81,25.4 27.81,23.75 28.96,22.61 31.75,22.61 33.02,23.88 | DA1.A 33.02,23.88 | 33.02,26.54 33.53,26.04 33.53,24.38 33.02,23.88
N$36
  Bottom 0.813: R10.1 D4.C D5.C D6.C
N$37
  Top 0.813: R10.2 58.42,24.13 55.92,26.63 RV4.E
N$38
  Top 0.813: IC3.9 43.05,5.08 44.2,6.22 44.2,12.7 | IC3.12 44.2,12.7 | 44.2,12.7 45.47,13.97 55.85,13.97 56.87,14.99 56.87,20.6 RV4.A 53.34,24.13 RV4.S
  Bottom 0.813: IC3.12 40.51,12.7 37.97,10.16 IC3.4 IC2.11
N$39
  Top 1.27: T3.E 78.74,29.21 81.28,26.67 R13.1
N$40
  Bottom 1.27: R13.2 86.4,24.09 RV1.E
N$41
  Top 0.813: R37.1 69.34,50.29 69.34,57.15 69.34,57.4 69.34,58.08 66.53,60.88 64.85,60.88 D12.A
  Bottom 0.813: R33.2 R36.1 61.47,46.99 62.74,48.26 64.77,48.26 R37.1
  Bottom 1.27: R37.1 71.1,46.99 72.93,48.82 74.73,48.82 76.2,50.29 76.2,53.23 81.28,58.3 81.28,71.12 78.74,73.66 T8.B
N$42
  Top 0.813: R38.1 68.17,54.2 68.17,57.56 D11.A
  Bottom 0.813: R30.2 R35.1 61.47,52.07 62.74,53.34 64.77,53.34 R38.1
  Bottom 1.27: R38.1 71.12,52.07 73.66,54.61 73.66,62.61 74.93,63.88 74.93,72.39 73.66,73.66 T7.B
N$43
  Top 1.27: D10.A R34.1
  Bottom 0.813: R24.2 R34.1 61.59,57.15 62.87,58.42 64.77,58.42 R39.1
  Bottom 1.27: R39.1 68.58,59.69 68.58,62.87 69.83,64.11 69.83,72.42 68.58,73.66 T6.B
N$44
  Top 1.27: T10.B 54.61,73.66 52.07,76.2 T9.C R28.1 R29.2
N$45
  Top 1.27: T10.E R32.1
N$46
  Top 2: RV5.S L4.2
N$47
  Top 2: RV6.S L5.2
N$48
  Top 2: RV7.S L6.2
N$49
  Bottom 1.27: R25.2 91.44,63.5 RV5.A
N$50
  Bottom 1.27: R26.2 83.82,59.69 RV6.A
N$51
  Bottom 1.27: R27.2 76.2,55.88 RV7.A
N$52
  Bottom 1.27: R45.2 78.78,62.19 RV6.E
N$53
  Bottom 1.27: R44.2 71.16,58.38 RV7.E
N$54  (via drill 0.35)
  Top 0.813: IC7.5 35.56,49.53 36.69,50.66 36.69,53.3 v36.66,53.34
  Bottom 0.813: v36.66,53.34 25.4,53.34 24.13,54.61 IC6.3
N$55  (via drill 0.35)
  Top 0.813: v37.95,47.02 37.95,48.26 39.37,49.69 39.37,55.88 40.64,57.15 IC7.13
  Bottom 0.813: IC6.6 24.13,46.99 25.4,45.72 36.32,45.72 37.62,47.02 v37.95,47.02
N$56
  Top 0.813: IC7.10 40.58,49.53 38.99,47.94 38.99,46.61 38.1,45.72 32.39,45.72 31.12,44.45 IC6.8
N$57  (via drill 0.35)
  Top 0.813: IC7.6 35.31,46.99 36.32,48.01 36.32,48.8 37.72,50.2 v37.72,53.34
  Bottom 0.813: v37.72,53.34 40.26,55.88 62.23,55.88 D7.A
N$58
  Bottom 0.813: D8.A 62.23,50.8 44.45,50.8 43.18,52.07 IC7.11
N$59
  Top 0.813: D9.A 62.23,48.26 45.72,48.26 44.45,46.99 44.45,45.72 43.18,44.45 IC7.8
N$60
  Top 0.813: IC5.2 IC5.13
N$61
  Top 0.813: IC5.4 IC5.11
N$62
  Top 0.813: IC5.6 IC5.9
N$63
  Top 1.27: IC5.12 R24.1
N$64
  Top 1.27: IC5.10 R30.1
N$65
  Top 1.27: IC5.8 R33.1
N$66
  Top 0.813: R36.2 D9.C
N$67
  Top 0.813: R35.2 D8.C
N$68
  Top 0.813: R34.2 D7.C
N$69
  Bottom 0.813: IC8.12 18.54,54.61 19.81,55.88 24.77,55.88 26.03,54.61 IC6.12
N$70  (via drill 0.35)
  Top 0.813: IC7.3 35.56,54.61 36.75,55.8 36.75,58.83 v37.31,59.38
  Bottom 0.813: v37.31,59.38 44.45,66.52 R40.2
N$71
  Top 0.813: R40.1 47.37,71.12 49.91,73.66 T9.B
N$72  (via drill 0.6)
  Top 1.27: V2.2 29.21,76.2 | 29.21,76.2 29.21,74.68 | 29.21,74.68 v29.21,72.39 | v29.21,72.39 V2.TAB | V2.TAB 28.07,72.97 28.07,73.53 29.21,74.68 | 29.21,76.2 30.43,74.98 30.43,72.67 29.59,71.83 V2.TAB | v29.21,72.39 28.07,71.25 28.07,70.36 | 28.07,70.36 28.07,68.58 | 28.07,68.58 28.07,67.44 | 27.43,67.31 R41.1 28.07,67.44 | 28.07,70.36 27.43,69.72 27.43,67.31 | 28.07,67.44 29.21,68.58 V2.TAB | V2.TAB 30.35,71.83 30.35,69.72 28.7,68.07 | 28.7,68.07 28.45,67.82 28.45,67.06 28.19,66.8 27.69,66.8 27.43,67.06 27.43,67.31 | 28.07,68.58 28.7,68.58 28.7,68.07
  Bottom 1.27: DA2.A 33.02,68.45 | 32.51,68.96 31.62,69.85 31.62,71.25 | 31.62,71.25 v30.48,72.39 | v30.48,72.39 v29.21,72.39 | v29.21,72.39 v27.94,72.39 | v27.94,72.39 27.43,71.88 27.43,68.33 27.81,67.94 27.81,67.31 | 27.81,67.31 R41.1 | R41.1 28.43,67.31 28.82,67.7 | 30.48,69.01 31.32,69.01 DA2.A | R41.1 27.94,70.74 29.21,72.01 v29.21,72.39 | v29.21,72.39 29.08,72.25 29.08,68.58 | 29.08,68.58 29.08,68.45 29.63,69.01 | 28.82,67.7 28.82,68.33 29.08,68.58 | v30.48,72.39 30.48,69.01 | 30.48,69.01 29.63,69.01 | 29.63,69.01 29.51,69.01 29.72,69.22 29.72,71.88 v29.21,72.39 | v30.48,72.39 30.48,73.66 | 30.48,73.66 29.97,74.17 28.45,74.17 27.94,73.66 | v27.94,72.39 27.94,73.66 | 27.94,73.66 30.48,73.66 | 31.62,71.25 32.51,70.36 32.51,68.96 | 32.51,68.96 33.02,68.45 | DA2.A 32.13,68.2 32.13,66.42 31.24,65.53 29.72,65.53 28.82,66.43 28.82,67.7 | 27.81,67.31 27.81,65.66 28.96,64.52 31.75,64.52 33.02,65.79 | DA2.A 33.02,65.79 | 33.02,68.45 33.53,67.94 33.53,66.29 33.02,65.79
N$73
  Top 0.813: V2.1 31.5,78 31.5,76.58 32.77,75.31 32.77,69.6 R41.2 30.48,66.42 29.21,65.15 26.67,65.15 25.4,66.42 R42.1
N$74
  Top 0.813: IC7.2 33.68,57.15 32.28,55.75 32.28,47.14 30.86,45.72 19.94,45.72 18.67,44.45 IC8.8
N$75  (via drill 0.35)
  Top 0.813: IC7.1 33.02,59.69 31.32,57.99 31.32,48.36 v31.22,48.26
  Bottom 0.813: IC8.6 11.43,46.99 12.7,45.72 17.78,45.72 20.32,48.26 v31.22,48.26
N$76
  Bottom 0.813: R43.1 D10.C D12.C D11.C
N$77
  Top 0.813: IC7.9 43.05,46.99 44.2,48.13 44.2,54.61 | IC7.12 44.2,54.61 | 44.2,54.61 45.47,55.88 55.85,55.88 56.87,56.9 56.87,62.51 RV8.A 53.34,66.04 RV8.S
  Bottom 0.813: IC7.12 40.51,54.61 37.97,52.07 IC7.4 IC6.11
N$78
  Top 1.27: T6.E 68.58,71.12 69.85,69.85 69.85,62.23 R44.1
N$79
  Top 1.27: R45.1 78.74,66.17 73.79,71.12 T7.E
N$80
  Top 1.27: T8.E 78.74,71.12 81.28,68.58 R46.1
N$81
  Bottom 1.27: R46.2 86.4,66 RV5.E
N$82
  Top 0.813: R43.2 58.42,66.04 55.92,68.54 RV8.E
N$176
  Top 1.27: T5.E R20.1
N$177
  Top 1.27: T5.B 54.61,31.75 52.07,34.29 T4.C R18.1 R19.2
R  (via drill 0.8)
  Top 2: v3.81,17.78 1.27,17.78
  Bottom 0.813: IC4.1 44.45,17.78 43.18,16.51 25.91,16.51 24.64,15.24 IC2.2 19.69,15.24 18.42,16.51 13.59,16.51 12.32,17.78 IC1.1 v3.81,17.78
  Bottom 2: 1.27,17.78 v3.81,17.78
R1  (via drill 0.8)
  Top 2: v3.81,59.69 1.27,59.69
  Bottom 0.813: IC5.1 44.45,59.69 43.18,58.42 25.91,58.42 24.64,57.15 IC6.2 19.69,57.15 18.42,58.42 13.59,58.42 12.32,59.69 IC8.1 v3.81,59.69
  Bottom 2: 1.27,59.69 v3.81,59.69
RED  (via drill 0.8)
  Top 1.8: v95.25,2.54 L3.1 C3.1
  Top 2: v95.25,2.54 97.79,2.54
  Bottom 1.8: v95.25,2.54 L3.1 C3.1
  Bottom 2: 97.79,2.54 v95.25,2.54
RED1  (via drill 0.8)
  Top 1.8: v95.25,44.45 L6.1 C11.1
  Top 2: v95.25,44.45 97.79,44.45
  Bottom 1.8: v95.25,44.45 L6.1 C11.1
  Bottom 2: 97.79,44.45 v95.25,44.45
S  (via drill 0.8)
  Top 2: 97.79,29.21 v95.25,29.21
  Bottom 1.8: R20.2 R21.1 62.23,35.69 63.37,36.83 86.36,36.83 88.9,34.29 88.9,30.48 90.17,29.21 v95.25,29.21
  Bottom 2: v95.25,29.21 97.79,29.21
S1  (via drill 0.8)
  Top 2: 97.79,71.12 v95.25,71.12
  Bottom 1.8: R32.2 R31.1 62.23,77.6 63.37,78.74 86.36,78.74 88.9,76.2 88.9,72.39 90.17,71.12 v95.25,71.12
  Bottom 2: v95.25,71.12 97.79,71.12
V  (via drill 0.8)
  Top 0.813: IC1.3 IC1.4 IC1.5
  Top 2: v3.81,7.62 1.27,7.62
  Bottom 0.813: IC1.5 v3.81,7.62
  Bottom 2: v3.81,7.62 1.27,7.62
V1  (via drill 0.8)
  Top 0.813: IC8.3 IC8.4 IC8.5
  Top 2: v3.81,49.53 1.27,49.53
  Bottom 0.813: IC8.5 v3.81,49.53
  Bottom 2: v3.81,49.53 1.27,49.53
VCC  (via drill 0.8)
  Top 1.27: 31.62,18.92 32.39,19.68 38.1,19.68 | 31.62,18.92 30.48,17.78 IC2.14 27.94,17.78 25.91,19.81 19.81,19.81 | 52.07,17.78 50.16,19.68 49.02,19.68 | 52.07,17.78 IC4.14 55.25,17.78 54.23,18.8 52.71,18.8 50.55,20.95 49.53,20.95 | 18.67,20.32 20.32,20.32 | 18.67,20.32 16.51,20.32 | 27.43,19.68 26.54,20.57 20.57,20.57 20.32,20.32 | 27.43,19.68 30.86,19.68 32.13,20.95 36.83,20.95 | 44.45,36.83 82.8,36.83 | 82.8,36.83 84.84,36.83 | 84.84,36.83 86.36,36.83 | 44.45,36.83 44.45,37.08 40.89,37.08 40.01,36.2 | 44.45,36.83 44.45,35.56 | 44.45,35.56 44.69,35.56 45.32,36.2 54.61,36.2 | 54.61,36.2 55.88,36.2 | 55.88,36.2 57.15,36.2 | 57.15,36.2 64.14,36.2 | 64.14,36.2 64.77,36.2 65.41,35.56 69.85,35.56 | T5.C 55.88,36.2 | T5.C 56.39,34.29 57.15,35.05 57.15,36.2 | T5.C 55.37,34.29 54.61,35.05 54.61,36.2 | 39.37,33.53 C5.+ 39.37,35.56 | 40.51,34.29 40.51,35.81 | 39.37,35.56 39.37,36.58 40.88,38.09 86.36,38.09 | 40.01,36.2 39.37,35.56 | 40.51,34.29 40.26,34.04 40.26,29.59 C6.1 | 40.51,34.29 41.21,34.99 | 44.45,35.56 41.21,35.56 41.21,34.99 | 39.5,29.21 39.37,29.21 39.37,33.53 | 39.5,29.21 C6.1 | 40.01,36.2 41.91,36.2 | 41.91,36.2 43.82,36.2 44.45,36.83 | 39.37,33.53 38.35,32.51 38.35,28.19 | C6.1 40.51,29.34 | C6.1 41.21,29.21 41.21,30.48 | 41.21,30.48 41.21,34.99 | 36.83,20.95 38.48,20.95 | 38.48,20.95 40.64,20.95 | 40.64,20.95 43.18,20.95 | 43.18,20.95 49.53,20.95 | 49.02,19.68 44.45,19.68 | 44.45,19.68 38.1,19.68 | 40.64,23.11 40.64,20.95 | C6.1 41.02,29.21 41.91,28.32 41.91,24.13 | 41.91,24.13 41.91,22.86 | 41.91,22.86 41.91,20.32 | 16.51,20.32 15.24,20.32 | 15.24,20.32 14.99,20.32 | 31.75,22.1 30.23,20.57 28.07,20.57 27.69,20.95 27.94,20.95 27.31,21.59
  Top 1.27: 49.53,20.95 48.39,22.1 43.94,22.1 41.91,24.13 | 14.99,20.32 13.97,21.34 13.97,19.05 15.24,17.78 IC1.14 | 22.73,21.59 27.31,21.59 | 13.97,21.59 14.61,22.23 | 14.61,22.23 14.86,22.48 15.88,22.48 14.35,24 | T2.C 71.12,34.29 69.85,35.56 | 74.93,35.56 73.66,34.29 | 74.93,35.56 76.2,34.29 T3.C 78.74,34.29 80.01,35.56 | 86.36,35.56 86.36,36.83 | 86.36,36.83 86.36,38.09 | 69.85,35.56 68.58,34.29 T1.C 66.04,34.29 64.14,36.2 | 69.85,35.56 74.93,35.56 | 74.93,35.56 80.01,35.56 | 86.36,38.09 93.99,38.09 v95.25,36.83 93.98,35.56 86.36,35.56 | 86.36,35.56 87.63,36.83 | 12.83,24 14.35,24 | 14.35,24 15.11,24 16.51,22.61 21.72,22.61 22.73,21.59 | 12.83,24 13.97,22.86 | 13.97,22.86 14.61,22.23 | 39.05,18.73 40.01,17.78 IC3.14 43.18,17.78 45.72,20.32 | 39.05,18.73 38.1,19.68 | 44.45,19.68 43.5,18.73 39.05,18.73 | 80.01,35.56 83.82,35.56 | 83.82,35.56 86.36,35.56 | 39.5,25.27 39.5,26.67 | 39.5,26.67 39.5,29.21 | 36.83,20.95 39.62,23.75 39.62,25.4 39.5,25.27 | 38.48,20.95 40.64,23.11 | C6.1 40.64,23.11 | 52.07,17.78 50.93,17.78 49.02,19.68 | 27.31,21.59 31.88,21.59 | IC1.14 16.51,20.32 | IC1.14 17.78,17.78 19.81,19.81 | 19.81,19.81 20.32,20.32 | 15.24,20.32 15.24,19.05 IC1.14 | IC1.14 16.51,18.16 18.67,20.32 | 44.45,35.56 R18.2 44.32,34.42 42.93,34.42 41.91,33.4 | 39.5,25.27 36.32,22.1 31.75,22.1 | 22.73,21.59 22.86,21.46 13.72,21.46 13.59,21.59 12.7,21.59 | 12.7,21.59 5.08,21.59 v3.81,22.86 | 12.7,21.59 13.97,20.32 14.99,20.32 | v3.81,22.86 4.95,24 12.83,24 | 13.97,22.86 v3.81,22.86 | 31.75,22.1 32.51,22.86 34.29,22.86 | 34.29,22.86 35.43,22.86 35.56,22.99 | 27.43,19.68 28.19,18.92 31.62,18.92 | 38.35,28.19 DA1.C 35.56,24.13 | 35.56,24.13 35.56,22.99
  Top 1.27: 35.56,24.13 34.29,22.86 | 38.35,28.19 38.35,26.92 35.56,24.13 | 39.5,26.67 35.81,22.99 35.56,22.99 | 41.91,22.86 43.18,21.59 43.18,20.95 | 41.91,36.2 41.91,33.4 | 41.91,33.4 41.91,31.18 41.21,30.48 | C4.+ 83.82,35.56 | C4.+ 82.8,34.04 82.8,36.83 | C4.+ 84.84,34.04 84.84,36.83
  Top 2: 86.36,36.83 87.63,36.83 v95.25,36.83 97.79,36.83 | 1.27,22.86 v3.81,22.86
  Bottom 1.27: 14.1,24 16,22.1 16.51,22.1 | 14.1,24 12.83,24 | 12.83,24 9.02,24 | 9.02,24 8.38,24 | 16.51,20.32 13.59,23.24 | 13.59,23.24 12.83,24 | 13.59,23.24 9.78,23.24 | 9.78,23.24 9.02,24 | 10.03,22.99 9.78,23.24 | 14.99,20.32 12.45,22.86 v3.81,22.86 | 16.51,20.32 15.88,20.32 | 15.88,20.32 14.99,20.32 | 16.51,20.32 17.02,20.32 17.02,18.29 IC1.14 | 16.51,22.61 15.11,24 14.1,24 | 9.53,22.86 8.38,24 | IC1.14 17.14,17.78 17.78,18.41 17.78,21.34 16.51,22.61 | IC1.14 15.88,17.78 | 15.88,17.78 14.99,18.67 14.99,20.32 | IC1.14 15.88,18.41 15.88,20.32 | v3.81,22.86 4.95,24 8.38,24 | v3.81,22.86 5.08,21.59 12.7,21.59 13.97,20.32 13.97,19.05 15.24,17.78 15.88,17.78 | 16.51,20.32 16.51,22.1 | 16.51,22.1 16.51,22.61
  Bottom 2: v3.81,22.86 1.27,22.86 | v95.25,36.83 97.79,36.83
VCC1  (via drill 0.8)
  Top 1.27: 31.62,60.83 32.39,61.59 38.1,61.59 | 31.62,60.83 30.48,59.69 IC6.14 27.94,59.69 25.91,61.72 19.81,61.72 | 52.07,59.69 50.16,61.59 49.02,61.59 | 52.07,59.69 IC5.14 55.25,59.69 54.23,60.71 52.71,60.71 50.55,62.87 49.53,62.87 | 18.67,62.23 20.32,62.23 | 18.67,62.23 16.51,62.23 | 27.43,61.59 26.54,62.48 20.57,62.48 20.32,62.23 | 27.43,61.59 30.86,61.59 32.13,62.87 36.83,62.87 | 44.45,78.74 82.8,78.74 | 82.8,78.74 84.84,78.74 | 84.84,78.74 86.36,78.74 | 44.45,78.74 44.45,78.99 40.89,78.99 40.01,78.11 | 44.45,78.74 44.45,77.47 | 44.45,77.47 44.69,77.47 45.32,78.11 54.61,78.11 | 54.61,78.11 55.88,78.11 | 55.88,78.11 57.15,78.11 | 57.15,78.11 64.14,78.11 | 64.14,78.11 64.77,78.11 65.41,77.47 69.85,77.47 | T10.C 55.88,78.11 | T10.C 56.39,76.2 57.15,76.96 57.15,78.11 | T10.C 55.37,76.2 54.61,76.96 54.61,78.11 | 39.37,75.44 C13.+ 39.37,77.47 | 40.51,76.2 40.51,77.72 | 39.37,77.47 39.37,78.49 40.88,80 86.36,80 | 40.01,78.11 39.37,77.47 | 40.51,76.2 40.26,75.95 40.26,71.5 C14.1 | 40.51,76.2 41.21,76.9 | 44.45,77.47 41.21,77.47 41.21,76.9 | 39.5,71.12 39.37,71.12 39.37,75.44 | 39.5,71.12 C14.1 | 40.01,78.11 41.91,78.11 | 41.91,78.11 43.82,78.11 44.45,78.74 | 39.37,75.44 38.35,74.42 38.35,70.1 | C14.1 40.51,71.25 | C14.1 41.21,71.12 41.21,72.39 | 41.21,72.39 41.21,76.9 | 36.83,62.87 38.48,62.87 | 38.48,62.87 40.64,62.87 | 40.64,62.87 43.18,62.87 | 43.18,62.87 49.53,62.87 | 49.02,61.59 44.45,61.59 | 44.45,61.59 38.1,61.59 | 40.64,65.02 40.64,62.87 | C14.1 41.02,71.12 41.91,70.23 41.91,66.04 | 41.91,66.04 41.91,64.77 | 41.91,64.77 41.91,62.23 | 16.51,62.23 15.24,62.23 | 15.24,62.23 14.99,62.23 | 31.75,64.01 30.23,62.48 28.07,62.48 27.69,62.87 27.94,62.87 27.31,63.5
  Top 1.27: 49.53,62.87 48.39,64.01 43.94,64.01 41.91,66.04 | 14.99,62.23 13.97,63.25 13.97,60.96 15.24,59.69 IC8.14 | 22.73,63.5 27.31,63.5 | 13.97,63.5 14.61,64.14 | 14.61,64.14 14.86,64.39 15.88,64.39 14.35,65.91 | T7.C 71.12,76.2 69.85,77.47 | 74.93,77.47 73.66,76.2 | 74.93,77.47 76.2,76.2 T8.C 78.74,76.2 80.01,77.47 | 86.36,77.47 86.36,78.74 | 86.36,78.74 86.36,80 | 69.85,77.47 68.58,76.2 T6.C 66.04,76.2 64.14,78.11 | 69.85,77.47 74.93,77.47 | 74.93,77.47 80.01,77.47 | 86.36,80 93.99,80 v95.25,78.74 93.98,77.47 86.36,77.47 | 86.36,77.47 87.63,78.74 | 12.83,65.91 14.35,65.91 | 14.35,65.91 15.11,65.91 16.51,64.52 21.72,64.52 22.73,63.5 | 12.83,65.91 13.97,64.77 | 13.97,64.77 14.61,64.14 | 39.05,60.64 40.01,59.69 IC7.14 43.18,59.69 45.72,62.23 | 39.05,60.64 38.1,61.59 | 44.45,61.59 43.5,60.64 39.05,60.64 | 80.01,77.47 83.82,77.47 | 83.82,77.47 86.36,77.47 | 39.5,67.18 39.5,68.58 | 39.5,68.58 39.5,71.12 | 36.83,62.87 39.62,65.66 39.62,67.31 39.5,67.18 | 38.48,62.87 40.64,65.02 | C14.1 40.64,65.02 | 52.07,59.69 50.93,59.69 49.02,61.59 | 27.31,63.5 31.88,63.5 | IC8.14 16.51,62.23 | IC8.14 17.78,59.69 19.81,61.72 | 19.81,61.72 20.32,62.23 | 15.24,62.23 15.24,60.96 IC8.14 | IC8.14 16.51,60.07 18.67,62.23 | 44.45,77.47 R28.2 44.32,76.33 42.93,76.33 41.91,75.31 | 39.5,67.18 36.32,64.01 31.75,64.01 | 22.73,63.5 22.86,63.37 13.72,63.37 13.59,63.5 12.7,63.5 | 12.7,63.5 5.08,63.5 v3.81,64.77 | 12.7,63.5 13.97,62.23 14.99,62.23 | v3.81,64.77 4.95,65.91 12.83,65.91 | 13.97,64.77 v3.81,64.77 | 31.75,64.01 32.51,64.77 34.29,64.77 | 34.29,64.77 35.43,64.77 35.56,64.9 | 27.43,61.59 28.19,60.83 31.62,60.83 | 38.35,70.1 DA2.C 35.56,66.04 | 35.56,66.04 35.56,64.9
  Top 1.27: 35.56,66.04 34.29,64.77 | 38.35,70.1 38.35,68.83 35.56,66.04 | 39.5,68.58 35.81,64.9 35.56,64.9 | 41.91,64.77 43.18,63.5 43.18,62.87 | 41.91,78.11 41.91,75.31 | 41.91,75.31 41.91,73.09 41.21,72.39 | C12.+ 83.82,77.47 | C12.+ 82.8,75.95 82.8,78.74 | C12.+ 84.84,75.95 84.84,78.74
  Top 2: 86.36,78.74 87.63,78.74 v95.25,78.74 97.79,78.74 | 1.27,64.77 v3.81,64.77
  Bottom 1.27: 14.1,65.91 16,64.01 16.51,64.01 | 14.1,65.91 12.83,65.91 | 12.83,65.91 9.02,65.91 | 9.02,65.91 8.38,65.91 | 16.51,62.23 13.59,65.15 | 13.59,65.15 12.83,65.91 | 13.59,65.15 9.78,65.15 | 9.78,65.15 9.02,65.91 | 10.03,64.9 9.78,65.15 | 14.99,62.23 12.45,64.77 v3.81,64.77 | 16.51,62.23 15.88,62.23 | 15.88,62.23 14.99,62.23 | 16.51,62.23 17.02,62.23 17.02,60.2 IC8.14 | 16.51,64.52 15.11,65.91 14.1,65.91 | 9.53,64.77 8.38,65.91 | IC8.14 17.14,59.69 17.78,60.33 17.78,63.25 16.51,64.52 | IC8.14 15.88,59.69 | 15.88,59.69 14.99,60.58 14.99,62.23 | IC8.14 15.88,60.33 15.88,62.23 | v3.81,64.77 4.95,65.91 8.38,65.91 | v3.81,64.77 5.08,63.5 12.7,63.5 13.97,62.23 13.97,60.96 15.24,59.69 15.88,59.69 | 16.51,62.23 16.51,64.01 | 16.51,64.01 16.51,64.52
  Bottom 2: v3.81,64.77 1.27,64.77 | v95.25,78.74 97.79,78.74
VIN
  Top 1.27: C7.1 22.86,30.48 | 22.86,30.48 22.86,31.11 | 22.86,31.11 22.86,31.62 22.73,31.75 | 22.86,30.48 23.75,30.48 | C7.1 22.86,29.84 | 23.75,30.48 23.75,29.21 | 22.86,29.72 C7.1 | DC_IN.1 13.64,33.02 | 13.64,33.02 18.8,33.02 | 18.8,33.02 C8.+ 21.46,33.02 | 22.23,32.26 21.46,33.02 | 22.23,32.26 14.15,32.26 DC_IN.1 | 22.86,31.11 21.59,31.11 | 19.94,31.37 21.59,31.37 21.59,31.11 | 19.94,31.37 16.64,31.37 | 16.64,31.37 14.02,31.37 DC_IN.1 | C7.1 21.59,30.48 21.59,31.11 | 18.8,33.02 17.91,33.91 14.22,33.91 13.64,33.33 13.64,33.02 | 19.94,31.37 22.1,29.21 23.75,29.21 | DC_IN.1 13.64,30.35 15.62,30.35 16.64,31.37 | 23.75,29.21 24.13,29.21 25.27,30.35 25.27,31.62 26.9,33.25 V1.3 26.77,36.25 26.64,36.25 25.78,35.38 25.78,34.29 | 23.75,30.48 24.13,30.86 24.13,31.75 | 24.13,31.75 25.4,33.02 | 25.4,33.02 25.78,33.4 25.78,34.29 | 22.23,32.26 22.73,31.75 | 22.73,31.75 24.13,31.75 | 21.46,33.02 24.51,33.02 | 24.51,33.02 25.4,33.02 | 25.78,34.29 24.51,33.02
  Bottom 1.27: DC_IN.1 13.64,33.2 14.35,33.91 17.91,33.91 18.8,33.02 C8.+ | DC_IN.1 13.64,30.55 13.84,30.35 15.62,30.35 16.69,31.42 | 16.69,31.42 20.02,31.42 20.14,31.29 | C7.1 22.23,29.21 21.27,30.16 | 20.14,31.29 21.27,30.16 | C7.1 24.13,29.21 24.89,29.97 24.89,32.26 24,33.15 20.45,33.15 C8.+ | DC_IN.1 15.04,33.15 20.19,33.15 C8.+ | DC_IN.1 14.02,32.13 17.78,32.13 17.91,32.26 23.62,32.26 23.75,32.13 | C7.1 23.88,30.23 | 23.75,32.13 23.88,32 23.88,30.23 | 23.88,30.23 21.34,30.23 21.27,30.16 | 23.75,32.13 22.91,31.29 20.14,31.29 | DC_IN.1 13.97,31.42 16.69,31.42
VIN1
  Top 1.27: C15.1 22.86,72.39 | 22.86,72.39 22.86,73.03 | 22.86,73.03 22.86,73.53 22.73,73.66 | 22.86,72.39 23.75,72.39 | C15.1 22.86,71.75 | 23.75,72.39 23.75,71.12 | 22.86,71.63 C15.1 | DC_IN1.1 13.64,74.93 | 13.64,74.93 18.8,74.93 | 18.8,74.93 C16.+ 21.46,74.93 | 22.23,74.17 21.46,74.93 | 22.23,74.17 14.15,74.17 DC_IN1.1 | 22.86,73.03 21.59,73.03 | 19.94,73.28 21.59,73.28 21.59,73.03 | 19.94,73.28 16.64,73.28 | 16.64,73.28 14.02,73.28 DC_IN1.1 | C15.1 21.59,72.39 21.59,73.03 | 18.8,74.93 17.91,75.82 14.22,75.82 13.64,75.24 13.64,74.93 | 19.94,73.28 22.1,71.12 23.75,71.12 | DC_IN1.1 13.64,72.26 15.62,72.26 16.64,73.28 | 23.75,71.12 24.13,71.12 25.27,72.26 25.27,73.53 26.9,75.16 V2.3 26.77,78.16 26.64,78.16 25.78,77.29 25.78,76.2 | 23.75,72.39 24.13,72.77 24.13,73.66 | 24.13,73.66 25.4,74.93 | 25.4,74.93 25.78,75.31 25.78,76.2 | 22.23,74.17 22.73,73.66 | 22.73,73.66 24.13,73.66 | 21.46,74.93 24.51,74.93 | 24.51,74.93 25.4,74.93 | 25.78,76.2 24.51,74.93
  Bottom 1.27: DC_IN1.1 13.64,75.11 14.35,75.82 17.91,75.82 18.8,74.93 C16.+ | DC_IN1.1 13.64,72.47 13.84,72.26 15.62,72.26 16.69,73.33 | 16.69,73.33 20.02,73.33 20.14,73.2 | C15.1 22.23,71.12 21.27,72.07 | 20.14,73.2 21.27,72.07 | C15.1 24.13,71.12 24.89,71.88 24.89,74.17 24,75.06 20.45,75.06 C16.+ | DC_IN1.1 15.04,75.06 20.19,75.06 C16.+ | DC_IN1.1 14.02,74.04 17.78,74.04 17.91,74.17 23.62,74.17 23.75,74.04 | C15.1 23.88,72.14 | 23.75,74.04 23.88,73.91 23.88,72.14 | 23.88,72.14 21.34,72.14 21.27,72.07 | 23.75,74.04 22.91,73.2 20.14,73.2 | DC_IN1.1 13.97,73.33 16.69,73.33
Y  (via drill 0.8)
  Top 0.813: 25.4,15.24 22.86,17.78 IC2.1 | IC2.9 27.94,5.08 26.03,6.99 26.03,9.53 25.4,10.16 | 25.4,15.24 25.4,10.16 | IC2.4 25.4,10.16 | IC2.13 25.4,15.24
  Top 2: v3.81,10.16 1.27,10.16
  Bottom 0.813: IC2.4 19.43,10.16 18.16,11.43 6.35,11.43 5.08,10.16 v3.81,10.16
  Bottom 2: 1.27,10.16 v3.81,10.16
Y1  (via drill 0.8)
  Top 0.813: 25.4,57.15 22.86,59.69 IC6.1 | IC6.9 27.94,46.99 26.03,48.9 26.03,51.44 25.4,52.07 | 25.4,57.15 25.4,52.07 | IC6.4 25.4,52.07 | IC6.13 25.4,57.15
  Top 2: v3.81,52.07 1.27,52.07
  Bottom 0.813: IC6.4 19.43,52.07 18.16,53.34 6.35,53.34 5.08,52.07 v3.81,52.07
  Bottom 2: 1.27,52.07 v3.81,52.07

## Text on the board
tPlace: + | - | S | + | TrueRGB | - | - | R | - | G | - | B | Y | B | V | G | H | - | R | + | - | S | + | TrueRGB | - | - | R | - | G | - | B | Y | B | V | G | H | - | R
bPlace: + | - | S | + | - | - | R | - | G | - | B | Y | B | V | G | H | - | R | + | - | S | + | - | - | R | - | G | - | B | Y | B | V | G | H | - | R
_tNames: DC_IN | C8 | C5 | R18 | T4 | T5 | R21 | T1 | T2 | T3 | C4 | R20 | R14 | V1 | R19 | C7 | C6 | R10 | D4 | D5 | D6 | R13 | R17 | R1 | R4 | D1 | R9 | R15 | R23 | R22 | DA1 | RV4 | R2 | R5 | D2 | R8 | R12 | RV1 | R3 | R6 | D3 | R7 | R11 | R16 | IC1 | IC2 | IC3 | IC4 | RV2 | RV3 | C1 | L1 | C2 | L2 | C3 | L3 | DC_IN | C8 | C5 | R18 | T4 | T5 | R21 | T1 | T2 | T3 | C4 | R20 | R14 | V1 | R19 | C7 | C6 | R10 | D4 | D5 | D6 | R13 | R17 | R1 | R4 | D1 | R9 | R15 | R23 | R22 | DA1 | RV4 | R2 | R5 | D2 | R8 | R12 | RV1 | R3 | R6 | D3 | R7 | R11 | R16 | IC1 | IC2 | IC3 | IC4 | RV2 | RV3 | C1 | L1 | C2 | L2 | C3 | L3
